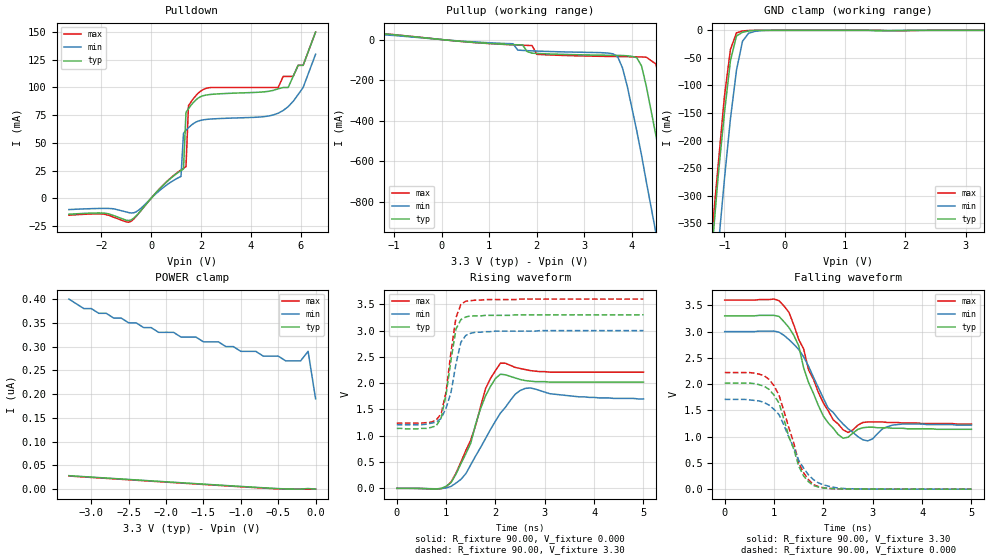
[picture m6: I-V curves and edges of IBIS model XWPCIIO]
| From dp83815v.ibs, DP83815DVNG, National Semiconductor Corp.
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|   Model XWPCIIO
[Model]   XWPCIIO
Model_type   I/O
Polarity   Non-Inverting
Enable   Active-High
Vinl =   0.80V
Vinh =   2.00V
Vmeas =   1.50V
Cref =  20.00pF
Rref = 100.00k
C_comp   7.00pF   7.00pF   7.00pF
[Temperature Range]   25.00   0.14k   0.000
[Voltage Range]   3.30V   3.00V   3.60V
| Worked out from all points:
|   slope of the pulldown table from 0 to 0.495 V, typ, clamps not added: 41.1 ohm
|   slope of the pullup table from 0 to 0.495 V, typ, clamps not added: 46.3 ohm
|   GND clamp passes 1 mA (typ) near -0.57 V on its own axis
|   rising waveform, R_fixture 90.00, V_fixture 0.000: 20-80 % time 473ps typ, 618ps min, 489ps max; typ from 0 V to 2.02 V
|   rising waveform, R_fixture 90.00, V_fixture 3.30: 20-80 % time 221ps typ, 254ps min, 212ps max; typ from 1.14 V to 3.3 V
|   falling waveform, R_fixture 90.00, V_fixture 3.30: 20-80 % time 478ps typ, 570ps min, 563ps max; typ from 3.3 V to 1.14 V
|   falling waveform, R_fixture 90.00, V_fixture 0.000: 20-80 % time 411ps typ, 518ps min, 425ps max; typ from 2.02 V to 0 V
[Pulldown]
| voltage   I(typ)   I(min)   I(max)
-3.3V     -14.39mA   -10.17mA   -15.24mA
-800mV    -19.53mA   -13.23mA   -20.76mA
1.2V      25.03mA    19.75mA    25.67mA
1.3V      26.44mA    58.68mA    27.18mA
1.4V      77.51mA    61.37mA    28.58mA
1.5V      80.9mA     63.71mA    83.57mA
1.9V      90.62mA    69.77mA    95.07mA
5.1V      98.82mA    76.8mA     100mA
5.5V      100mA      82.72mA    110mA
5.9V      120mA      93.63mA    120mA
6.1V      120mA      100mA      120mA
6.6V      150mA      130mA      150mA
[Pullup]
| voltage   I(typ)   I(min)   I(max)
-3.3V     1.71mA     1.39mA     1.85mA
-2.1V     42.44mA    6.83mA     45.52mA
3.6V      -77.76mA   -70.33mA   -83.5mA
3.8V      -78.64mA   -140mA     -84.19mA
4.1V      -89.52mA   -450mA     -85.13mA
4.3V      -230mA     -700mA     -86.88mA
4.5V      -470mA     -950mA     -120mA
4.7V      -720mA     -1.21A     -320mA
4.9V      -980mA     -1.47A     -570mA
5.1V      -1.25A     -1.74A     -830mA
5.3V      -1.52A     -2A        -1.1A
6.6V      -3.27A     -3.74A     -2.85A
[GND_clamp]
| voltage   I(typ)   I(min)   I(max)
-3.3V     -3.17A     -3.25A     -3.15A
-1.2V     -390mA     -510mA     -360mA
-1.1V     -260mA     -390mA     -240mA
-1V       -150mA     -270mA     -120mA
-900mV    -54.84mA   -160mA     -34.62mA
-800mV    -10.25mA   -72.25mA   -4.59mA
-700mV    -3.49mA    -19.74mA   -1.22mA
-600mV    -1.27mA    -5.32mA    -220uA
-500mV    -240uA     -1.99mA    -19.49uA
-200mV    -54.35nA   -13.64uA   -1.12nA
3.3V      130pA      270nA      34.78pA
[POWER_clamp]
| voltage   I(typ)   I(min)   I(max)
-3.3V     28.42nA    400nA      27.71nA
-3.1V     26.43nA    380nA      25.72nA
-2.8V     23.45nA    370nA      22.75nA
-2.1V     16.53nA    330nA      15.83nA
-1.9V     14.56nA    330nA      13.86nA
-1.3V     8.69nA     310nA      7.99nA
-1V       5.8nA      290nA      5.1nA
-800mV    3.91nA     290nA      3.21nA
-400mV    540pA      270nA      140pA
-200mV    160pA      270nA      180pA
-100mV    1.41nA     290nA      44.74pA
0V        130pA      190nA      38.86pA
[Ramp]
| variable   typ   min   max
dV/dt_r   1.82/0.39n   1.62/0.52n   1.99/0.39n
dV/dt_f   1.84/0.47n   1.64/0.57n   2.00/0.48n
R_load = 0.50k
[Rising Waveform]
R_fixture = 90.00
V_fixture = 0.000
V_fixture_min = 0.000
V_fixture_max = 0.000
| time   V(typ)   V(min)   V(max)
0s        36.47uV    36.37uV    39.57uV
900ps     65.91uV    -5mV       -7.26mV
1.1ns     110mV      37.71mV    120mV
1.5ns     860mV      450mV      920mV
1.8ns     1.76V      950mV      1.9V
2.1ns     2.17V      1.43V      2.38V
2.4ns     2.1V       1.79V      2.3V
2.7ns     2.04V      1.91V      2.24V
3.7ns     2.02V      1.74V      2.21V
5ns       2.02V      1.7V       2.21V
[Rising Waveform]
R_fixture = 90.00
V_fixture = 3.30
V_fixture_min = 3.00
V_fixture_max = 3.60
| time   V(typ)   V(min)   V(max)
0s        1.14V      1.21V      1.24V
700ps     1.16V      1.24V      1.26V
900ps     1.34V      1.33V      1.42V
1ns       1.79V      1.53V      1.84V
1.1ns     2.45V      1.83V      2.6V
1.2ns     3.03V      2.37V      3.25V
1.3ns     3.21V      2.78V      3.5V
1.4ns     3.26V      2.91V      3.56V
2ns       3.29V      2.99V      3.59V
5ns       3.3V       3V         3.6V
[Falling Waveform]
R_fixture = 90.00
V_fixture = 3.30
V_fixture_min = 3.00
V_fixture_max = 3.60
| time   V(typ)   V(min)   V(max)
0s        3.3V       3V         3.6V
1ns       3.31V      3.01V      3.62V
1.2ns     3.19V      2.93V      3.49V
1.5ns     2.73V      2.66V      2.85V
1.7ns     2.03V      2.34V      2.27V
2ns       1.39V      1.73V      1.64V
2.5ns     990mV      1.15V      1.08V
2.9ns     1.18V      920mV      1.28V
3.4ns     1.16V      1.22V      1.27V
5ns       1.14V      1.22V      1.24V
[Falling Waveform]
R_fixture = 90.00
V_fixture = 0.000
V_fixture_min = 0.000
V_fixture_max = 0.000
| time   V(typ)   V(min)   V(max)
0s        2.02V      1.71V      2.22V
600ps     2.01V      1.69V      2.21V
900ps     1.9V       1.6V       2.09V
1.1ns     1.64V      1.42V      1.79V
1.4ns     760mV      790mV      880mV
1.5ns     440mV      550mV      500mV
1.6ns     250mV      400mV      310mV
1.8ns     68.5mV     180mV      86.46mV
2.4ns     4.73mV     13.83mV    5.07mV
5ns       140uV      250uV      170uV
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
